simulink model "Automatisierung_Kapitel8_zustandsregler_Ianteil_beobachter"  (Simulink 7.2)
settings: Solver=ode45  StartTime=0.0  StopTime=100  MaxStep=0.2  RelTol=1e-3
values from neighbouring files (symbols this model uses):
  Ac = [0,1,0,0;-1,-1,1,1;0,0,0,1;0.1,0.1,-0.2,-0.2]    [Automatisierung_Kapitel8.m]
  AdL = Ad+kbeo'*cc    [Automatisierung_Kapitel8.m]
  Bc = [bc,bvc]    [Automatisierung_Kapitel8.m]
  BdL = [bd,-kbeo']    [Automatisierung_Kapitel8.m]
  Cc = eye(4)    [Automatisierung_Kapitel8.m]
  CdL = eye(4)    [Automatisierung_Kapitel8.m]
  Dc = [0,0;0,0;0,0;0,0]    [Automatisierung_Kapitel8.m]
  DdL = [0,0;0,0;0,0;0,0]    [Automatisierung_Kapitel8.m]
  kI = ke(5)    [Automatisierung_Kapitel8.m]
  kP = 1/(cc*inv(eye(4)-Ad)*bd)    [Automatisierung_Kapitel8.m]
  kx = kP*cc+ke(1:4)    [Automatisierung_Kapitel8.m]
  Ta = 2    [Automatisierung_Kapitel8.m]
libraries: simulink x1

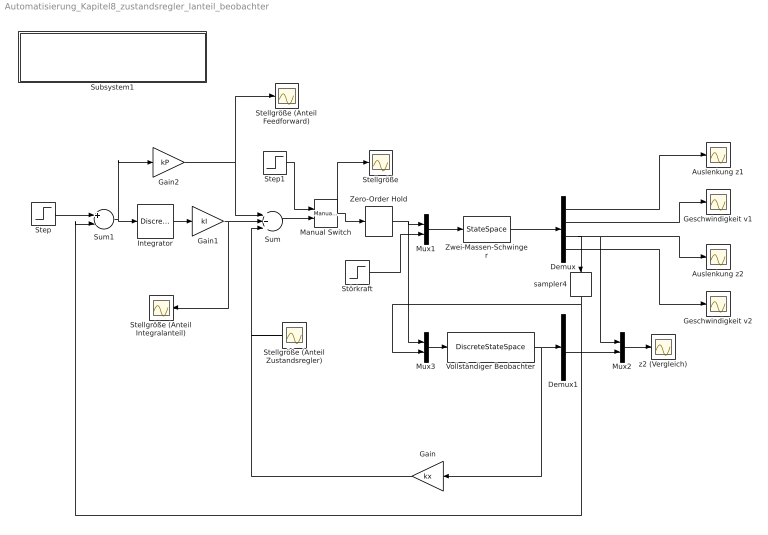
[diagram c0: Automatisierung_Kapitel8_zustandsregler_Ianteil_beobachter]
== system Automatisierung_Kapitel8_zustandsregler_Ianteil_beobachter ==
  Auslenkung z1 : Scope
  Auslenkung z2 : Scope
  Demux : Demux
  Demux1 : Demux
  Gain : Gain  Orientation=left  Gain=kx  Multiplication=Matrix(K*u)  ParameterDataType=sfix(16)  ParameterScaling=2^0  OutDataType=sfix(16)  OutScaling=2^0
  Gain1 : Gain  Gain=kI  ParameterDataType=sfix(16)  ParameterScaling=2^0  OutDataType=sfix(16)  OutScaling=2^0
  Gain2 : Gain  Gain=kP  ParameterDataType=sfix(16)  ParameterScaling=2^0  OutDataType=sfix(16)  OutScaling=2^0
  Geschwindigkeit v1 : Scope
  Geschwindigkeit v2 : Scope
  Integrator : DiscreteTransferFcn  Denominator=[1 -1]  SampleTime=Ta
  Manual Switch : simulink/Signal Routing/Manual Switch  SystemSampleTime=-1  sw=0  action=0  varsize=off
  Mux1 : Mux  Inputs=2
  Mux2 : Mux  Inputs=2
  Mux3 : Mux  Inputs=2
  Stellgröße : Scope
  Stellgröße (Anteil Feedforward) : Scope
  Stellgröße (Anteil Integralanteil) : Scope
  Stellgröße (Anteil Zustandsregler) : Scope
  Step : Step  Time=0  SampleTime=0
  Step1 : Step  Time=0  SampleTime=0
  Störkraft : Step  Time=20  SampleTime=0
  Subsystem1 : Subsystem
  Sum : Sum  Inputs=+++  OutDataType=sfix(16)  OutScaling=2^0
  Sum1 : Sum  Inputs=+-  OutDataType=sfix(16)  OutScaling=2^0
  Vollständiger Beobachter : DiscreteStateSpace  A=AdL  B=BdL  C=CdL  D=DdL  X0=[0,0,0,0]  SampleTime=Ta
  Zero-Order Hold : ZeroOrderHold  SampleTime=Ta
  Zwei-Massen-Schwinger : StateSpace  A=Ac  B=Bc  C=Cc  D=Dc  X0=[0,0,0,0]
  sampler4 : DiscreteTransferFcn  Orientation=down  Denominator=[1]  SampleTime=Ta
  z2 (Vergleich) : Scope
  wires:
  Zwei-Massen-Schwinger/1 -> Demux/1
  Mux1/1 -> Zwei-Massen-Schwinger/1
  Zero-Order Hold/1 -> Mux1/1, Mux3/1
  Störkraft/1 -> Mux1/2
  Demux/1 -> Auslenkung z1/1
  Demux/3 -> sampler4/1, Auslenkung z2/1, Mux2/1
  Demux/2 -> Geschwindigkeit v1/1
  Demux/4 -> Geschwindigkeit v2/1
  Gain2/1 -> Sum/1, Stellgröße (Anteil Feedforward)/1
  Sum/1 -> Manual Switch/2
  Manual Switch/1 -> Zero-Order Hold/1, Stellgröße/1
  Step1/1 -> Manual Switch/1
  Step/1 -> Sum1/1
  Sum1/1 -> Integrator/1, Gain2/1
  Gain/1 -> Sum/3, Stellgröße (Anteil Zustandsregler)/1
  Integrator/1 -> Gain1/1
  Gain1/1 -> Sum/2, Stellgröße (Anteil Integralanteil)/1
  Mux3/1 -> Vollständiger Beobachter/1
  Vollständiger Beobachter/1 -> Gain/1, Demux1/1
  sampler4/1 -> Mux3/2, Sum1/2
  Demux1/3 -> Mux2/2
  Mux2/1 -> z2 (Vergleich)/1

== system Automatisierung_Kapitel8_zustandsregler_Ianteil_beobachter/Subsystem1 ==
